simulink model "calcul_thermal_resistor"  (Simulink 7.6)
settings: Solver=ode15s  StartTime=0.0  StopTime=0.4  RelTol=1e-3
InitFcn:
  | clc
  | clear all
  | close all
  | 
  | Vcc=12;
  | R=1e3;
StopFcn:
  | load Temp_Rth.mat
  | plotyy(x(1,:),x(2,:), x(1,:),x(3,:))
  | grid
  | title('Tension aux bornes de R et résistance de la thermistance')
  | xlabel('temps')
  | 
  | delete *.mat
libraries: fl_lib x17, nesl_utility x5, elec_lib x2

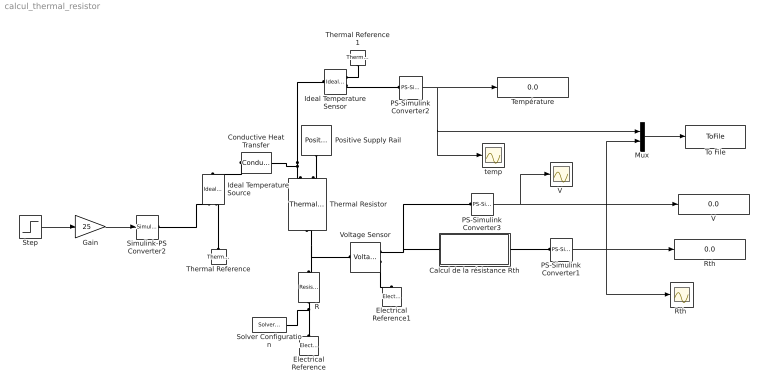
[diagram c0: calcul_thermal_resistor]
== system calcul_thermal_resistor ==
  Calcul de la résistance Rth : Subsystem
  Conductive Heat Transfer : fl_lib/Thermal/Thermal Elements/Conductive Heat Transfer  DialogController=NetworkEngine.DynNeDlgSource  SystemSampleTime=-1  area=1e-04 m^2  thickness=0.1 m  th_cond=401 W/(m*K)  Q_Log=off  T_Log=off  LocalVarNames=|Q|T  LocalVarDescs=|Q|T  LocalVarLogging=[0 0]
  Electrical Reference : fl_lib/Electrical/Electrical Elements/Electrical Reference  DialogController=NetworkEngine.DynNeDlgSource  SystemSampleTime=-1  i_Log=off  LocalVarNames=|i  LocalVarDescs=|i  LocalVarLogging=[]
  Electrical Reference1 : fl_lib/Electrical/Electrical Elements/Electrical Reference  DialogController=NetworkEngine.DynNeDlgSource  SystemSampleTime=-1  i_Log=off  LocalVarNames=|i  LocalVarDescs=|i  LocalVarLogging=[]
  Gain : Gain  Gain=25
  Ideal Temperature Sensor : fl_lib/Thermal/Thermal Sensors/Ideal Temperature Sensor  DialogController=NetworkEngine.DynNeDlgSource  SystemSampleTime=-1  Qs_Log=off  Ts_Log=off  LocalVarNames=|Qs|Ts  LocalVarDescs=|Qs|Ts  LocalVarLogging=[0 0]
  Ideal Temperature Source : fl_lib/Thermal/Thermal Sources/Ideal Temperature Source  DialogController=NetworkEngine.DynNeDlgSource  SystemSampleTime=-1  Q_Log=off  T_Log=off  LocalVarNames=|Q|T  LocalVarDescs=|Q|T  LocalVarLogging=[0 0]
  Mux : Mux  Inputs=2
  PS-Simulink Converter1 : nesl_utility/PS-Simulink Converter  DialogController=NetworkEngine.DynNeUtilDlgSource  SystemSampleTime=-1  PhysicalDomain=network_engine_domain  LeftPortType=input  RightPortType=output  SubClassName=ps_output  Unit=V  AffineConversion=off
  PS-Simulink Converter2 : nesl_utility/PS-Simulink Converter  DialogController=NetworkEngine.DynNeUtilDlgSource  SystemSampleTime=-1  PhysicalDomain=network_engine_domain  LeftPortType=input  RightPortType=output  SubClassName=ps_output  Unit=1  AffineConversion=off
  PS-Simulink Converter3 : nesl_utility/PS-Simulink Converter  DialogController=NetworkEngine.DynNeUtilDlgSource  SystemSampleTime=-1  PhysicalDomain=network_engine_domain  LeftPortType=input  RightPortType=output  SubClassName=ps_output  Unit=V  AffineConversion=off
  Positive Supply Rail : elec_lib/Sources/Positive Supply Rail  DialogController=NetworkEngine.DynNeDlgSource  SystemSampleTime=-1  v0=Vcc V  current_Log=off  voltage_Log=off  power_Log=off  LocalVarNames=|current|voltage|power  LocalVarDescs=|Current (A)|Voltage (V)|Power (W)  LocalVarLogging=[0 0 0]
  R : fl_lib/Electrical/Electrical Elements/Resistor  DialogController=NetworkEngine.DynNeDlgSource  SystemSampleTime=-1  R=R Ohm  i_Log=off  v_Log=off  LocalVarNames=|current|voltage|power  LocalVarDescs=|Resistor current (A)|Voltage across resistor (V)|Power (W)  LocalVarLogging=[0 0 0]
  Rth : Display
  "Rth " : Scope
  Simulink-PS Converter2 : nesl_utility/Simulink-PS Converter  DialogController=NetworkEngine.DynNeUtilDlgSource  SystemSampleTime=-1  PhysicalDomain=network_engine_domain  LeftPortType=input  RightPortType=output  SubClassName=ps_input  Unit=1  AffineConversion=off  InputFilterTimeConstant=.001  UdotUserProvided=0
  Solver Configuration : nesl_utility/Solver Configuration  DialogController=NetworkEngine.DynNeUtilDlgSource  SystemSampleTime=-1  PhysicalDomain=network_engine_domain  LeftPortType=input  RightPortType=generic  SubClassName=solver  Accelerate=off  Profile=off  ResidualTolerance=1e-9  MaxNonlinIter=12  MaxModeIter=2  DoFixedCost=off  UseLocalSampling=off  DoDC=off  LinearAlgebra=Sparse  LocalSolverSampleTime=.001  LocalSolverChoice=NE_BACKWARD_EULER_ADVANCER  UseLocalSolver=off
  Step : Step  Time=0  SampleTime=0
  Température : Display
  Thermal Reference : fl_lib/Thermal/Thermal Elements/Thermal Reference  DialogController=NetworkEngine.DynNeDlgSource  SystemSampleTime=-1  Q_Log=off  LocalVarNames=|Q  LocalVarDescs=|Q  LocalVarLogging=0
  Thermal Reference1 : fl_lib/Thermal/Thermal Elements/Thermal Reference  DialogController=NetworkEngine.DynNeDlgSource  SystemSampleTime=-1  Q_Log=off  LocalVarNames=|Q  LocalVarDescs=|Q  LocalVarLogging=0
  Thermal Resistor : elec_lib/Passive Devices/Thermal Resistor  DialogController=NetworkEngine.DynNeDlgSource  SystemSampleTime=-1  R0=1 Ohm  T0=25 C  alpha=5e-05 1/K  tc=10 s  K_d=0.001 W/K  init_temp=25 C  current_Log=off  voltage_Log=off  power_Log=off  temperature_Log=off  heat_flow_Log=off  LocalVarNames=|current|voltage|power|temperature|heat_flow  LocalVarDescs=|Resistor current (A)|Voltage across resistor (V)|Power (W)|Themistor temperature (K)|Heat flow (J/s)  LocalVarLogging=[0 0 0 0 0]
  To File : ToFile  Filename=Temp_Rth  MatrixName=x
  V : Display
  "V " : Scope
  Voltage Sensor : fl_lib/Electrical/Electrical Sensors/Voltage Sensor  DialogController=NetworkEngine.DynNeDlgSource  SystemSampleTime=-1  i1_Log=off  v1_Log=off  LocalVarNames=|i1|v1  LocalVarDescs=|i1|v1  LocalVarLogging=[]
  temp : Scope
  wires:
  Step/1 -> Gain/1
  Gain/1 -> Simulink-PS Converter2/1
  PS-Simulink Converter1/1 -> "Rth "/1, Rth/1, Mux/2
  PS-Simulink Converter2/1 -> Température/1, temp/1, Mux/1
  PS-Simulink Converter3/1 -> "V "/1, V/1
  Mux/1 -> To File/1
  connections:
  Positive Supply Rail/RConn1 -- Thermal Resistor/LConn2
  Thermal Resistor/RConn1 -- R/RConn1 -- Voltage Sensor/LConn1
  R/LConn1 -- Electrical Reference/LConn1 -- Solver Configuration/RConn1
  Voltage Sensor/RConn2 -- Electrical Reference1/LConn1
  Thermal Reference/LConn1 -- Ideal Temperature Source/RConn2
  Simulink-PS Converter2/RConn1 -- Ideal Temperature Source/RConn1
  Conductive Heat Transfer/LConn1 -- Ideal Temperature Source/LConn1
  Thermal Reference1/LConn1 -- Ideal Temperature Sensor/RConn1
  Ideal Temperature Sensor/RConn2 -- PS-Simulink Converter2/LConn1
  Calcul de la résistance Rth/RConn1 -- PS-Simulink Converter1/LConn1
  Voltage Sensor/RConn1 -- Calcul de la résistance Rth/LConn1 -- PS-Simulink Converter3/LConn1
  Thermal Resistor/LConn1 -- Conductive Heat Transfer/RConn1 -- Ideal Temperature Sensor/LConn1

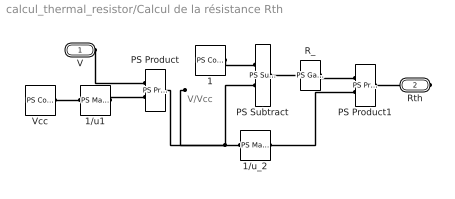
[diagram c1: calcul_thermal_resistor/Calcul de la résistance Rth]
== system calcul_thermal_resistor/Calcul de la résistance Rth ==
  note: V/Vcc
  1 : fl_lib/Physical Signals/Sources/PS Constant  DialogController=NetworkEngine.DynNeDlgSource  SystemSampleTime=-1  constant=1  LocalVarLogging=[]
  1/u1 : fl_lib/Physical Signals/Functions/PS Math Function  DialogController=NetworkEngine.DynNeDlgSource  SystemSampleTime=-1  fcn_choice=9  LocalVarLogging=[]
  1/u_2 : fl_lib/Physical Signals/Functions/PS Math Function  DialogController=NetworkEngine.DynNeDlgSource  SystemSampleTime=-1  fcn_choice=9  LocalVarLogging=[]
  PS Product : fl_lib/Physical Signals/Functions/PS Product  DialogController=NetworkEngine.DynNeDlgSource  SystemSampleTime=-1  LocalVarLogging=[]
  PS Product1 : fl_lib/Physical Signals/Functions/PS Product  DialogController=NetworkEngine.DynNeDlgSource  SystemSampleTime=-1  LocalVarLogging=[]
  PS Subtract : fl_lib/Physical Signals/Functions/PS Subtract  DialogController=NetworkEngine.DynNeDlgSource  SystemSampleTime=-1  LocalVarLogging=[]
  R_ : fl_lib/Physical Signals/Functions/PS Gain  DialogController=NetworkEngine.DynNeDlgSource  SystemSampleTime=-1  gain=R  LocalVarLogging=[]
  Vcc : fl_lib/Physical Signals/Sources/PS Constant  DialogController=NetworkEngine.DynNeDlgSource  SystemSampleTime=-1  constant=Vcc  LocalVarLogging=[]
  V : PMIOPort  Port=1  Side=Left
  Rth : PMIOPort  Port=2  Side=Right
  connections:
  1/RConn1 -- PS Subtract/LConn1
  Vcc/RConn1 -- 1/u1/LConn1
  1/u1/RConn1 -- PS Product/LConn2
  1/u_2/LConn1 -- PS Subtract/LConn2 -- PS Product/RConn1
  1/u_2/RConn1 -- PS Product1/LConn2
  R_/RConn1 -- PS Product1/LConn1
  PS Subtract/RConn1 -- R_/LConn1
  V/RConn1 -- PS Product/LConn1
  Rth/RConn1 -- PS Product1/RConn1
